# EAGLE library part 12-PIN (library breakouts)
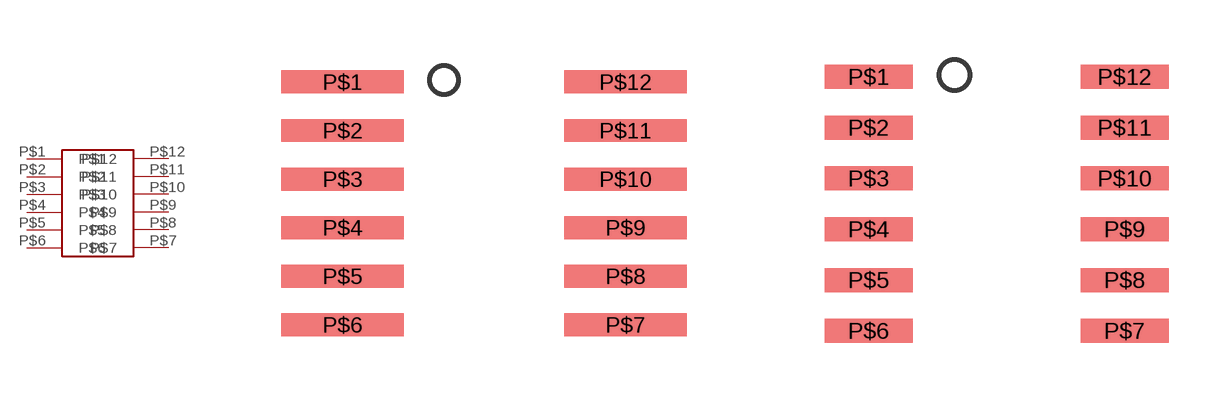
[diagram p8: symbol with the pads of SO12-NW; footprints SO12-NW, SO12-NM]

Designator prefix -

## 12-PINSOIC-NW  [SO12-NW]
P$1  P$1
P$2  P$2
P$3  P$3
P$4  P$4
P$5  P$5
P$6  P$6
P$7  P$7
P$8  P$8
P$9  P$9
P$10  P$10
P$11  P$11
P$12  P$12

## 12-PINSOIC-NM  [SO12-NM]
Pads as for SO12-NW

## 12-PINSOIC-M  [SO12-M]
Pads as for SO12-NW

## 12-PINTSSOP-N  [TSSOP12-3.9]
Pads as for SO12-NW

## 12-PINSOIC-N  [SO12-N]
Pads as for SO12-NW

## 12-PINSOIC-MW  [SO12-MW]
Pads as for SO12-NW

## 12-PINSOIC-W  [SO12-W]
Pads as for SO12-NW

## 12-PINTSSOP-W  [TSSOP12-5.3]
Pads as for SO12-NW

## 12-PINTSSOP-NW  [TSSOP12-NW]
Pads as for SO12-NW

## Footprint SO12-NW (pad centres in mm)
smd 3.2 x 0.6: P$1 -3.7,3.175; P$2 -3.7,1.905; P$3 -3.7,0.635; P$4 -3.7,-0.635; P$5 -3.7,-1.905; P$6 -3.7,-3.175; P$7 3.7,-3.175; P$8 3.7,-1.905; P$9 3.7,-0.635; P$10 3.7,0.635; P$11 3.7,1.905; P$12 3.7,3.175

## Footprint SO12-NM (pad centres in mm)
smd 2.2 x 0.6: P$1 -3.2,3.175; P$2 -3.2,1.905; P$3 -3.2,0.635; P$4 -3.2,-0.635; P$5 -3.2,-1.905; P$6 -3.2,-3.175; P$7 3.2,-3.175; P$8 3.2,-1.905; P$9 3.2,-0.635; P$10 3.2,0.635; P$11 3.2,1.905; P$12 3.2,3.175

## Footprint SO12-M (pad centres in mm)
smd 1.2 x 0.6: P$1 -3.7,3.175; P$2 -3.7,1.905; P$3 -3.7,0.635; P$4 -3.7,-0.635; P$5 -3.7,-1.905; P$6 -3.7,-3.175; P$7 3.7,-3.175; P$8 3.7,-1.905; P$9 3.7,-0.635; P$10 3.7,0.635; P$11 3.7,1.905; P$12 3.7,3.175

## Footprint TSSOP12-3.9 (pad centres in mm)
smd 1.4 x 0.35: P$1 -2.65,1.625; P$2 -2.65,0.975; P$3 -2.65,0.325; P$4 -2.65,-0.325; P$5 -2.65,-0.975; P$6 -2.65,-1.625; P$7 2.65,-1.625; P$8 2.65,-0.975; P$9 2.65,-0.325; P$10 2.65,0.325; P$11 2.65,0.975; P$12 2.65,1.625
